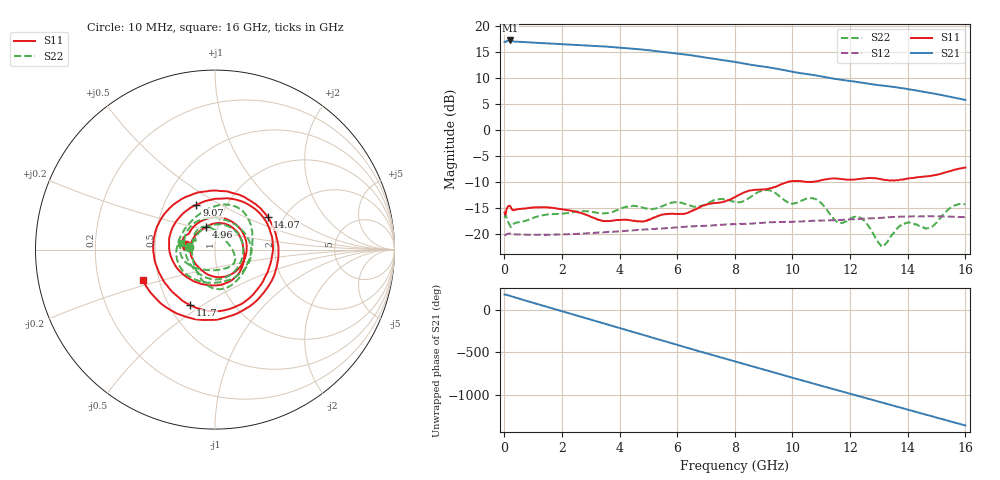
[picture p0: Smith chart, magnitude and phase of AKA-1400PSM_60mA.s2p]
!Keysight Technologies,P9375A,MY57211602,A.15.55.08
!Date: Tuesday, April 18, 2023 17:02:40
!Correction: S11(Cdelta 2-Port  )
!S21(Cdelta 2-Port  )
!S12(Cdelta 2-Port  )
!S22(Cdelta 2-Port  )
!S2P File: Measurements: S11, S21, S12, S22:
# Hz S  dB  R 50
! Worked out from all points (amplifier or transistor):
!   1600 points, 10 MHz to 16 GHz, reference 50 ohm
!   highest |S21| = 17.2 dB at 200 MHz (marker M1)
!   |S21| within 3 dB of that: start of sweep to 6.671 GHz
!   unconditionally stable (mu >= 1): start of sweep to end of sweep
!   at 2.67 GHz: K = 1.07, MAG = 16.4 dB, |S12| = -19.9 dB
!   at 8.01 GHz: K = 1.13, MAG = 13.4 dB, |S12| = -18.0 dB
!   at 16 GHz: K = 1.58, MAG = 6.7 dB, |S12| = -16.7 dB
!   S11 on the Smith chart (normalised r, x): 10 MHz: 0.72, +0.04; 4.96 GHz: 0.88, +0.23; 9.07 GHz: 0.72, +0.39; 11.7 GHz: 0.64, -0.45; 14.07 GHz: 1.65, +0.69; 16 GHz: 0.40, -0.17
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1e7  -15.81 171.6  16.91 175.6  -20.01 -4.1  -16.84 174.4
2e8  -14.56 158.5  17.15 159.4  -19.83 -17.1  -18.38 155.3
9e8  -14.91 89.9  16.77 89.0  -20.08 -75.0  -17.08 89.1
1.64e9  -14.89 19.0  16.55 15.6  -20.06 -135.6  -16.12 19.6
2.1e9  -15.27 -21.6  16.42 -29.8  -19.97 -173.5  -15.98 -24.7
2.68e9  -15.93 -71.7  16.26 -87.2  -19.84 138.8  -15.58 -75.5
3.24e9  -17.13 -117.1  16.08 -142.6  -19.65 92.4  -15.85 -121.3
3.69e9  -17.41 -149.5  15.91 172.8  -19.51 54.9  -15.77 -162.3
4.36e9  -17.28 154.9  15.61 106.6  -19.25 -1.3  -14.60 141.7
4.96e9  -17.32 110.6  15.31 47.3  -19.00 -51.5  -15.05 88.9
5.34e9  -16.45 79.7  15.06 9.8  -18.90 -83.7  -14.87 47.7
6.41e9  -15.75 -7.3  14.37 -95.3  -18.49 -174.7  -14.38 -52.1
7.2e9  -14.08 -76.1  13.68 -172.5  -18.30 117.5  -13.67 -135.1
8.01e9  -12.81 -146.4  13.03 108.9  -18.05 48.0  -13.77 155.8
9.07e9  -11.38 112.5  12.09 7.7  -17.75 -42.5  -11.50 62.7
9.89e9  -9.88 40.7  11.28 -70.6  -17.58 -113.4  -13.98 -7.5
1.067e10  -9.94 -27.1  10.58 -143.8  -17.41 180.0  -13.05 -81.6
1.17e10  -9.41 -113.9  9.62 119.4  -17.20 91.2  -17.82 177.3
1.334e10  -9.66 101.2  8.37 -33.8  -16.70 -51.2  -20.98 9.0
1.407e10  -9.24 32.0  7.77 -102.4  -16.58 -115.2  -17.73 -38.9
1.493e10  -8.65 -56.3  6.95 177.3  -16.55 169.3  -18.11 -114.3
1.6e10  -7.18 -157.4  5.76 78.8  -16.69 76.2  -14.24 169.2
